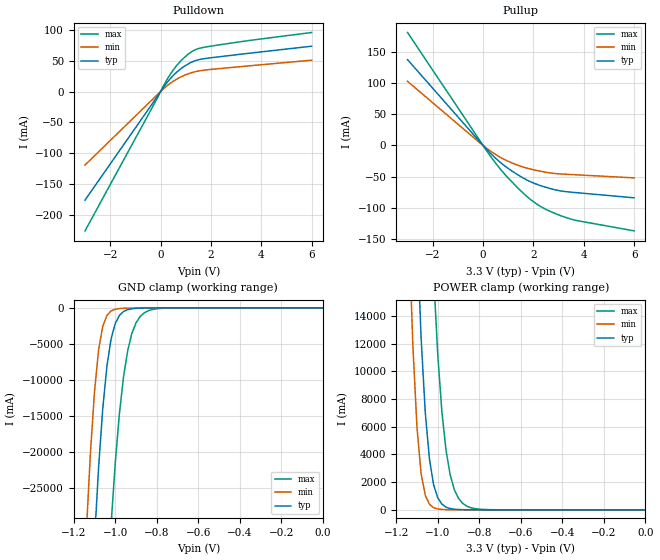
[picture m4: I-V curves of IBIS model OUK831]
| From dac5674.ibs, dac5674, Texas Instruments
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[Model]   OUK831
Model_type   3-state
Enable   Active-Low
Polarity   Non-Inverting
| signals   A, GZ, Y
Vmeas = 1.5
|   typ   min   max
C_comp   2.0965p   2.0088p   2.3774p
|   typ   min   max
[Temperature Range]   25   -40.0   125
|   typ   min   max
[Voltage Range]   3.30V   3.00V   3.60V
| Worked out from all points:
|   slope of the pulldown table from 0 to 0.495 V, typ, clamps not added: 19.3 ohm
|   slope of the pullup table from 0 to 0.495 V, typ, clamps not added: 24.2 ohm
|   GND clamp passes 1 mA (typ) near -0.58 V on its own axis
|   POWER clamp passes 1 mA (typ) near -0.64 V on its own axis
[Pulldown]
|   Voltage   I(typ)   I(min)   I(max)
-3V       -175.9mA   -119.1mA   -225.8mA
-200mV    -12.18mA   -7.956mA   -16.01mA
200mV     11.61mA    7.405mA    15.55mA
400mV     21.52mA    13.77mA    28.85mA
600mV     29.89mA    19.16mA    40.1mA
1V        42.47mA    27.25mA    57.28mA
1.3V      48.84mA    31.34mA    66.22mA
1.7V      53.08mA    34.51mA    71.52mA
3.6V      62.5mA     41.98mA    83.19mA
6V        73.47mA    50.83mA    95.74mA
[GND_clamp]
|   Voltage   I(typ)   I(min)   I(max)
-1.2V     -102.7A    -74.41A    -154.1A
-1.14V    -57.55A    -31.62A    -106.7A
-1.1V     -32.35A    -11.69A    -77.65A
-1.08V    -22.13A    -5.816A    -64.19A
-1.06V    -13.97A    -2.559A    -51.65A
-1.04V    -8.085A    -1.052A    -40.23A
-1.02V    -4.316A    -431.8mA   -30.14A
-980mV    -1.059A    -97.69mA   -14.73A
-960mV    -513.4mA   -60.94mA   -9.568A
-920mV    -131.1mA   -37.25mA   -3.566A
-880mV    -45.19mA   -28.49mA   -1.203A
0V        -130.5pA   -109.2pA   -2.072nA
[Pullup]
|   Voltage   I(typ)   I(min)   I(max)
-3V       138.1mA    103.2mA    181.7mA
-200mV    9.146mA    6.727mA    12.21mA
300mV     -12.88mA   -9.22mA    -17.63mA
900mV     -34.12mA   -23.64mA   -48.03mA
1.7V      -54.7mA    -36.06mA   -80.58mA
2.1V      -62.01mA   -39.98mA   -93.36mA
2.4V      -66.16mA   -42.43mA   -100.8mA
2.9V      -71.73mA   -45.34mA   -110.1mA
3.3V      -74.37mA   -46.38mA   -116.1mA
3.8V      -76.3mA    -47.46mA   -121.4mA
6V        -84.26mA   -52.21mA   -137.4mA
[POWER_clamp]
|   Voltage   I(typ)   I(min)   I(max)
-1.2V     83.43A     59.64A     127.8A
-1.14V    41.42A     20.8A      82.7A
-1.12V    29.85A     11.95A     68.94A
-1.1V     20.06A     5.958A     56.04A
-1.08V    12.41A     2.607A     44.19A
-1.06V    7.027A     1.048A     33.6A
-1.04V    3.679A     406.1mA    24.47A
-1.02V    1.819A     157.9mA    16.99A
-960mV    192.4mA    15.59mA    4.285A
-920mV    44.41mA    7.991mA    1.453A
-880mV    12.4mA     6.125mA    468.3mA
0V        154.5pA    161.2pA    3.029nA
[Ramp]
|   I(typ)   I(min)   I(max)
dV/dt_r   1.267/1.474n   0.957/2.769n   1.564/0.824n
dV/dt_f   1.332/1.513n   0.961/2.653n   1.616/0.826n
